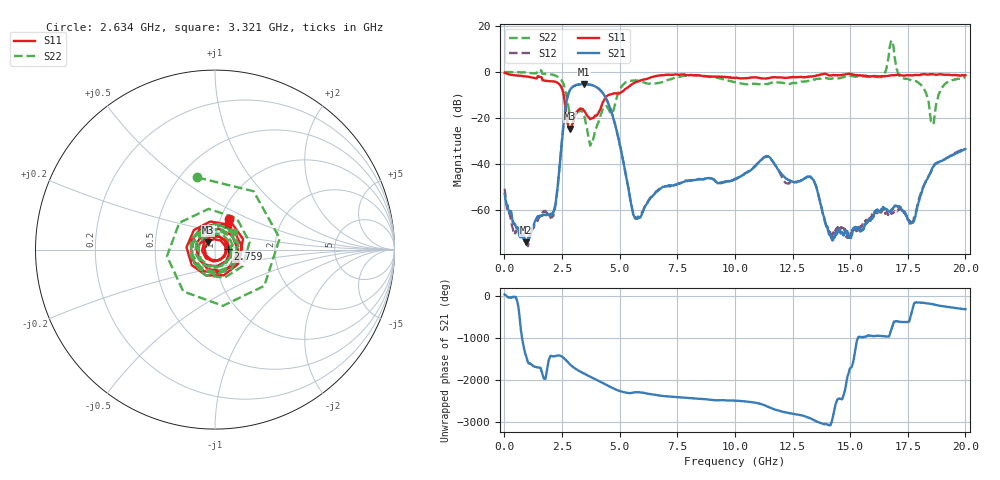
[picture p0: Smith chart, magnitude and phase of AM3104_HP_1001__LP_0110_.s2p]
!Created with skrf (http://scikit-rf.org).
# Hz S RI R 50.0
!freq ReS11 ImS11 ReS21 ImS21 ReS12 ImS12 ReS22 ImS22
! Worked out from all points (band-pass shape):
!   1601 points, 10 MHz to 20 GHz, reference 50 ohm
!   highest |S21| = -5.27 dB at 3.446 GHz (marker M1); lowest = -74.0 dB at 947 MHz (marker M2)
!   |S21| within 3 dB of the highest: 2.827 GHz to 4.198 GHz (1.371 GHz wide, 39 % of centre)
!   lowest |S11| = -24.7 dB at 2.834 GHz (marker M3), VSWR 1.12, Z = 45.9 + j3.77 ohm
!   |S11| at or under -10 dB: 2.571 GHz to 4.529 GHz (1.958 GHz wide, 55.2 % of centre)
!   |S22| runs from -32.0 to 13.6 dB; largest |S21 - S12| = 0.03
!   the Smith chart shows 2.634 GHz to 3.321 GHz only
!   S11 on the Smith chart (normalised r, x): 2.634 GHz: 1.09, +0.39; 2.759 GHz: 1.15, +0.01; 3.321 GHz: 1.11, +0.32
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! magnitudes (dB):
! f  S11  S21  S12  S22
! 10 MHz  -0.4  -53.0  -50.7  -0.1
! 947 MHz  -2.0  -74.0  -75.1  -0.2
! 2.134 GHz  -4.1  -60.8  -62.1  -1.4
! 2.634 GHz  -14.5  -17.1  -17.0  -7.7
! 2.759 GHz  -23.1  -10.2  -10.2  -14.1
! 2.834 GHz  -24.7  -8.1  -8.2  -18.2
! 3.321 GHz  -16.0  -5.4  -5.4  -16.8
! 3.346 GHz  -16.0  -5.3  -5.4  -16.8
! 3.446 GHz  -16.7  -5.3  -5.3  -19.1
! 3.771 GHz  -20.3  -5.7  -5.7  -31.2
! 4.545 GHz  -10.0  -14.6  -14.7  -16.8
! 5.67 GHz  -4.6  -63.1  -63.7  -3.7
! 6.682 GHz  -1.6  -51.5  -51.2  -4.9
! 10.01 GHz  -2.7  -46.6  -46.8  -4.6
! 11.39 GHz  -2.9  -36.6  -36.8  -5.3
! 13.34 GHz  -2.1  -46.3  -46.1  -3.6
! 14.24 GHz  -1.3  -72.8  -70.7  -2.8
! 16.68 GHz  -1.6  -60.6  -62.2  7.2
! 17.69 GHz  -1.6  -65.6  -65.4  -3.8
! 18.56 GHz  -0.9  -41.9  -42.1  -22.4
! 19.03 GHz  -1.2  -38.4  -38.3  -6.3
! 20 GHz  -1.4  -33.6  -33.1  -2.5
